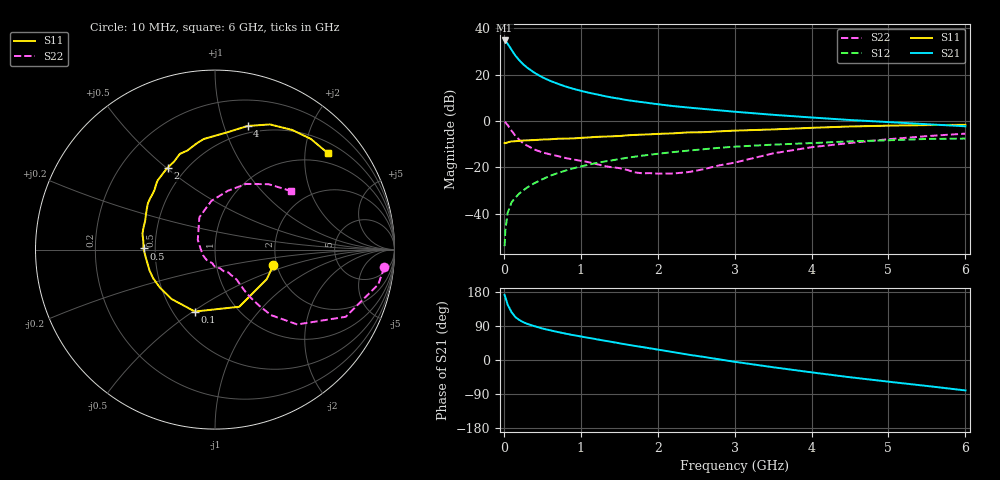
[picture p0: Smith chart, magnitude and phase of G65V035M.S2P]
! SIEMENS Small Signal Semiconductors
! BFG193
! Si NPN RF Bipolar Junction Transistor in SOT223
! VCE = 5 V  IC = 35 mA
! Common Emitter S-Parameters:  August  1996
# GHz  S  MA  R  50
!  f  S11  S21  S12  S22
! GHz  MAG  ANG  MAG  ANG  MAG  ANG  MAG  ANG
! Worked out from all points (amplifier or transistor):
!   36 points, 10 MHz to 6 GHz, reference 50 ohm
!   highest |S21| = 34.7 dB at 10 MHz (marker M1)
!   |S21| within 3 dB of that: start of sweep to 80.08 MHz
!   unconditionally stable (mu >= 1): 548.1 MHz to 2.338 GHz
!   at 250 MHz: K = 0.86, MSG = 27.2 dB, |S12| = -30.0 dB
!   at 1.4 GHz: K = 1.05, MAG = 12.3 dB, |S12| = -17.0 dB
!   at 6 GHz: K = 0.89, MSG = 2.7 dB, |S12| = -7.6 dB
!   S11 on the Smith chart (normalised r, x): 10 MHz: 1.91, -0.38; 100 MHz: 0.64, -0.51; 500 MHz: 0.43, +0.01; 2 GHz: 0.40, +0.50; 4 GHz: 0.43, +1.20; 6 GHz: 0.74, +2.51
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0.01  0.3363 -15.1  54.48 171.9  0.002 86.9  0.9487 -5.9
0.02  0.3322 -29.7  52.8 165.3  0.0045 80.8  0.9302 -12.0
0.05  0.3459 -67.0  46.16 145.8  0.0105 73.3  0.8189 -27.2
0.1  0.3628 -108.0  34.24 126.2  0.0176 65.9  0.6197 -42.3
0.15  0.3664 -131.2  25.67 113.2  0.0222 63.5  0.4799 -49.5
0.2  0.373 -145.3  20.47 105.8  0.0273 64.8  0.3955 -51.8
0.25  0.3795 -154.8  16.79 100.0  0.0317 64.5  0.3328 -53.4
0.3  0.3829 -161.9  14.27 95.7  0.0365 65.9  0.2961 -54.2
0.4  0.3882 -173.3  10.91 89.2  0.0458 66.8  0.2417 -54.3
0.5  0.3983 179.1  8.764 83.2  0.0554 66.2  0.2103 -54.1
0.6  0.403 172.8  7.375 78.5  0.0657 65.4  0.1914 -54.9
0.8  0.4168 162.7  5.553 69.7  0.085 62.8  0.1594 -58.5
1.1  0.4416 149.5  4.084 58.5  0.114 58.2  0.1295 -68.1
1.6  0.4899 132.0  2.823 40.6  0.1609 47.9  0.0884 -94.6
2  0.5267 120.1  2.301 27.5  0.1963 39.1  0.0732 -136.3
2.2  0.5412 114.8  2.096 20.8  0.2136 34.6  0.0737 -153.9
2.8  0.5984 100.2  1.696 1.7  0.2639 20.9  0.1104 150.3
3.5  0.6577 83.9  1.359 -19.1  0.3092 3.8  0.2003 115.8
4  0.7124 75.2  1.19 -32.6  0.3335 -5.9  0.2723 94.2
4.5  0.7617 66.3  1.05 -45.5  0.3643 -16.1  0.3352 77.7
5.5  0.8158 49.1  0.852 -68.5  0.4104 -39.4  0.4715 50.6
6  0.8269 40.6  0.769 -80.3  0.4169 -52.8  0.5341 37.7
